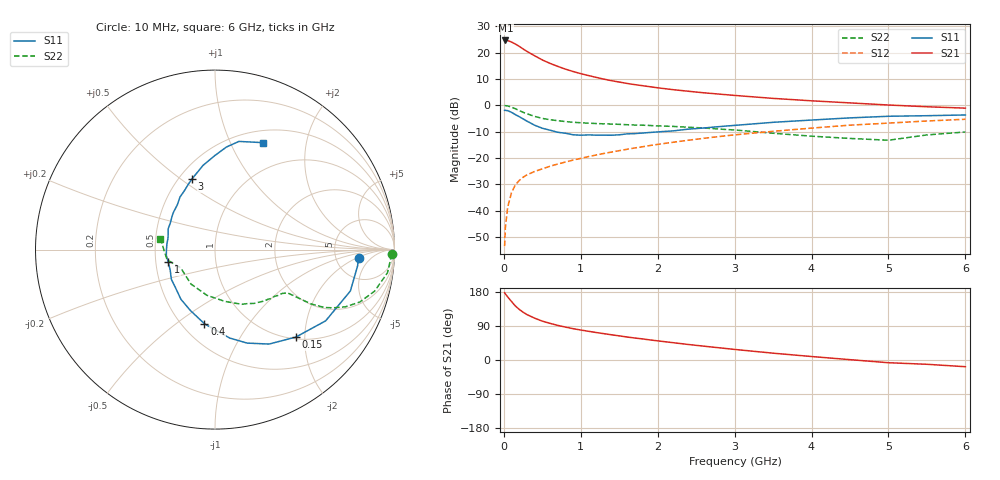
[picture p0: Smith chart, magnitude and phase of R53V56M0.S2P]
! SIEMENS Small Signal Semiconductors
! BFR183
! Si NPN RF Bipolar Junction Transistor in SOT23
! VCE = 3.5 V  IC = 6 mA
! Common Emitter S-Parameters:  May  1996
# GHz  S  MA  R  50
!  f  S11  S21  S12  S22
! GHz  MAG  ANG  MAG  ANG  MAG  ANG  MAG  ANG
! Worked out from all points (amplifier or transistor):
!   36 points, 10 MHz to 6 GHz, reference 50 ohm
!   highest |S21| = 24.6 dB at 20 MHz (marker M1)
!   |S21| within 3 dB of that: start of sweep to 238.4 MHz
!   unconditionally stable (mu >= 1): 944.5 MHz to 2.608 GHz
!   at 250 MHz: K = 0.47, MSG = 24.4 dB, |S12| = -27.4 dB
!   at 1.4 GHz: K = 1.06, MAG = 12.0 dB, |S12| = -17.8 dB
!   at 6 GHz: K = 0.88, MSG = 2.1 dB, |S12| = -5.3 dB
!   lowest NFmin = 1.20 dB at 450 MHz
!   S11 on the Smith chart (normalised r, x): 10 MHz: 8.46, -2.25; 150 MHz: 1.04, -1.80; 400 MHz: 0.64, -0.64; 1 GHz: 0.58, -0.09; 3 GHz: 0.58, +0.55; 6 GHz: 0.64, +1.34
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0.01  0.8013 -3.4  17 177.4  0.0021 88.1  0.9882 -1.5
0.02  0.7994 -6.6  17.02 174.3  0.0048 88.4  0.9801 -3.1
0.05  0.7887 -17.0  16.97 166.5  0.0116 82.5  0.9693 -7.7
0.1  0.7332 -32.8  15.88 154.3  0.0219 73.8  0.9188 -14.6
0.15  0.6634 -47.3  14.55 142.5  0.0307 68.0  0.8582 -19.9
0.2  0.6064 -60.2  13.18 133.6  0.0372 63.9  0.7933 -23.7
0.25  0.551 -71.0  11.73 126.2  0.0428 61.1  0.7346 -26.2
0.3  0.4994 -80.6  10.56 119.9  0.0475 59.4  0.69 -27.9
0.4  0.4174 -98.1  8.719 110.4  0.0552 57.9  0.6142 -29.5
0.5  0.3656 -112.1  7.261 102.6  0.0619 57.7  0.5623 -29.9
0.6  0.3356 -124.5  6.242 96.7  0.0694 57.9  0.5314 -30.2
0.8  0.2941 -145.8  4.859 86.9  0.0833 58.8  0.49 -30.6
1  0.2695 -165.4  3.982 79.1  0.0978 60.1  0.4648 -31.3
1.1  0.2733 -173.2  3.666 75.8  0.1057 60.5  0.4564 -32.2
1.3  0.2699 173.1  3.136 69.5  0.1213 60.6  0.4434 -33.8
1.6  0.2856 155.9  2.598 60.7  0.1455 60.2  0.4265 -37.3
2.2  0.3256 130.2  1.977 45.7  0.198 57.5  0.3963 -46.4
3  0.4142 108.0  1.537 27.9  0.2738 50.6  0.3393 -63.9
3.5  0.4738 98.1  1.35 18.0  0.3196 44.9  0.2937 -79.2
4.5  0.5753 83.6  1.108 0.9  0.4186 33.0  0.2339 -125.0
5.5  0.6329 71.2  0.936 -11.3  0.5023 20.7  0.273 -168.0
6  0.6538 65.7  0.881 -17.7  0.5416 12.7  0.3105 168.6
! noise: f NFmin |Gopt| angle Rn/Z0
0.45  1.2  0.21  41  0.24
0.9  1.25  0.24  101  0.21
1.8  2  0.32  175  0.14
